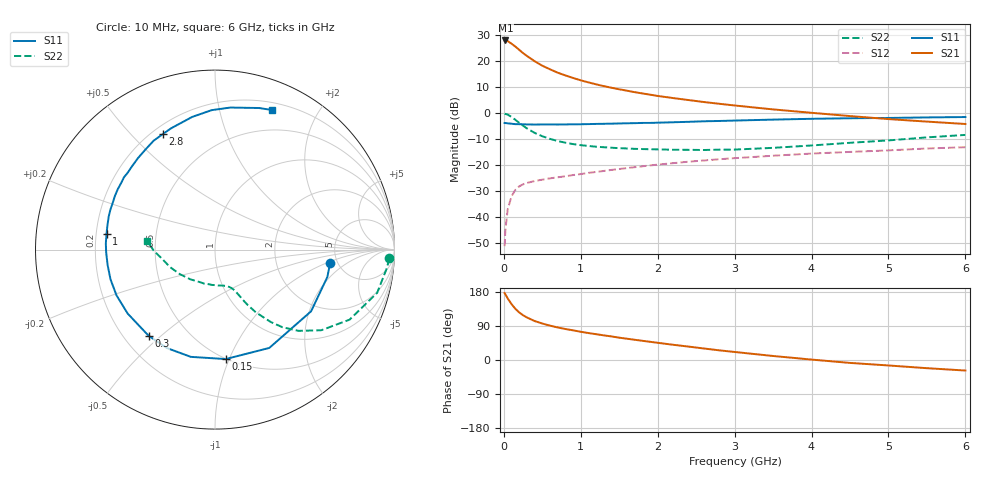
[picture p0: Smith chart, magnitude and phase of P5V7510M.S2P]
! SIEMENS Small Signal Semiconductors
! BFP183
! Si NPN RF Bipolar Junction Transistor in SOT143
! VCE = 0.75 V  IC = 10 mA
! Common Emitter S-Parameters:  March  1996
# GHz  S  MA  R  50
!  f  S11  S21  S12  S22
! GHz  MAG  ANG  MAG  ANG  MAG  ANG  MAG  ANG
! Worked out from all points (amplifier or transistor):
!   36 points, 10 MHz to 6 GHz, reference 50 ohm
!   highest |S21| = 27.9 dB at 20 MHz (marker M1)
!   |S21| within 3 dB of that: start of sweep to 175.7 MHz
!   unconditionally stable (mu >= 1): 964.8 MHz to end of sweep
!   at 250 MHz: K = 0.36, MSG = 25.2 dB, |S12| = -27.3 dB
!   at 1.4 GHz: K = 1.16, MAG = 13.4 dB, |S12| = -21.8 dB
!   at 6 GHz: K = 1.05, MAG = 3.0 dB, |S12| = -13.1 dB
!   S11 on the Smith chart (normalised r, x): 10 MHz: 4.35, -1.11; 150 MHz: 0.50, -0.97; 300 MHz: 0.30, -0.46; 1 GHz: 0.24, +0.07; 2.8 GHz: 0.24, +0.62; 6 GHz: 0.27, +1.45
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0.01  0.646 -6.6  24.68 176.7  0.0028 83.9  0.9719 -2.9
0.02  0.6443 -13.7  24.74 173.3  0.0057 83.5  0.9636 -6.0
0.05  0.6362 -32.7  24.07 162.5  0.0142 76.9  0.9352 -14.9
0.1  0.6258 -61.1  21.45 147.5  0.0254 62.9  0.8454 -27.5
0.15  0.6128 -84.4  18.85 135.0  0.0337 54.8  0.7431 -37.2
0.2  0.6126 -102.7  16.35 125.5  0.0394 48.9  0.6494 -44.2
0.25  0.6105 -116.1  14.15 118.1  0.043 44.2  0.5732 -49.0
0.3  0.6061 -127.6  12.48 112.3  0.0457 41.4  0.509 -52.4
0.4  0.6031 -143.8  9.905 102.8  0.0497 38.2  0.4179 -56.9
0.5  0.6051 -155.1  8.111 96.2  0.0529 37.1  0.3596 -59.4
0.6  0.6053 -164.1  6.924 90.7  0.056 36.9  0.3201 -61.0
0.7  0.6044 -171.7  5.958 85.9  0.0587 37.4  0.2911 -62.1
0.8  0.6063 -178.1  5.279 81.8  0.0613 37.7  0.2703 -63.2
1  0.6109 171.6  4.251 74.5  0.0676 38.7  0.2428 -65.4
1.1  0.6149 166.7  3.882 71.1  0.0713 39.2  0.2339 -66.7
1.5  0.6327 151.8  2.863 58.9  0.0846 40.2  0.2124 -72.7
2.2  0.6668 129.9  1.943 40.2  0.1096 38.4  0.1981 -89.3
2.8  0.7061 114.4  1.509 25.5  0.1302 34.6  0.1989 -107.1
3.5  0.7499 99.8  1.177 10.6  0.1522 29.9  0.2155 -129.9
4.5  0.7959 83.9  0.877 -7.7  0.18 21.7  0.2693 -158.9
5.5  0.8262 72.7  0.687 -21.6  0.2094 14.5  0.3421 -179.1
6  0.84 67.8  0.618 -27.8  0.2216 10.0  0.3814 172.4
